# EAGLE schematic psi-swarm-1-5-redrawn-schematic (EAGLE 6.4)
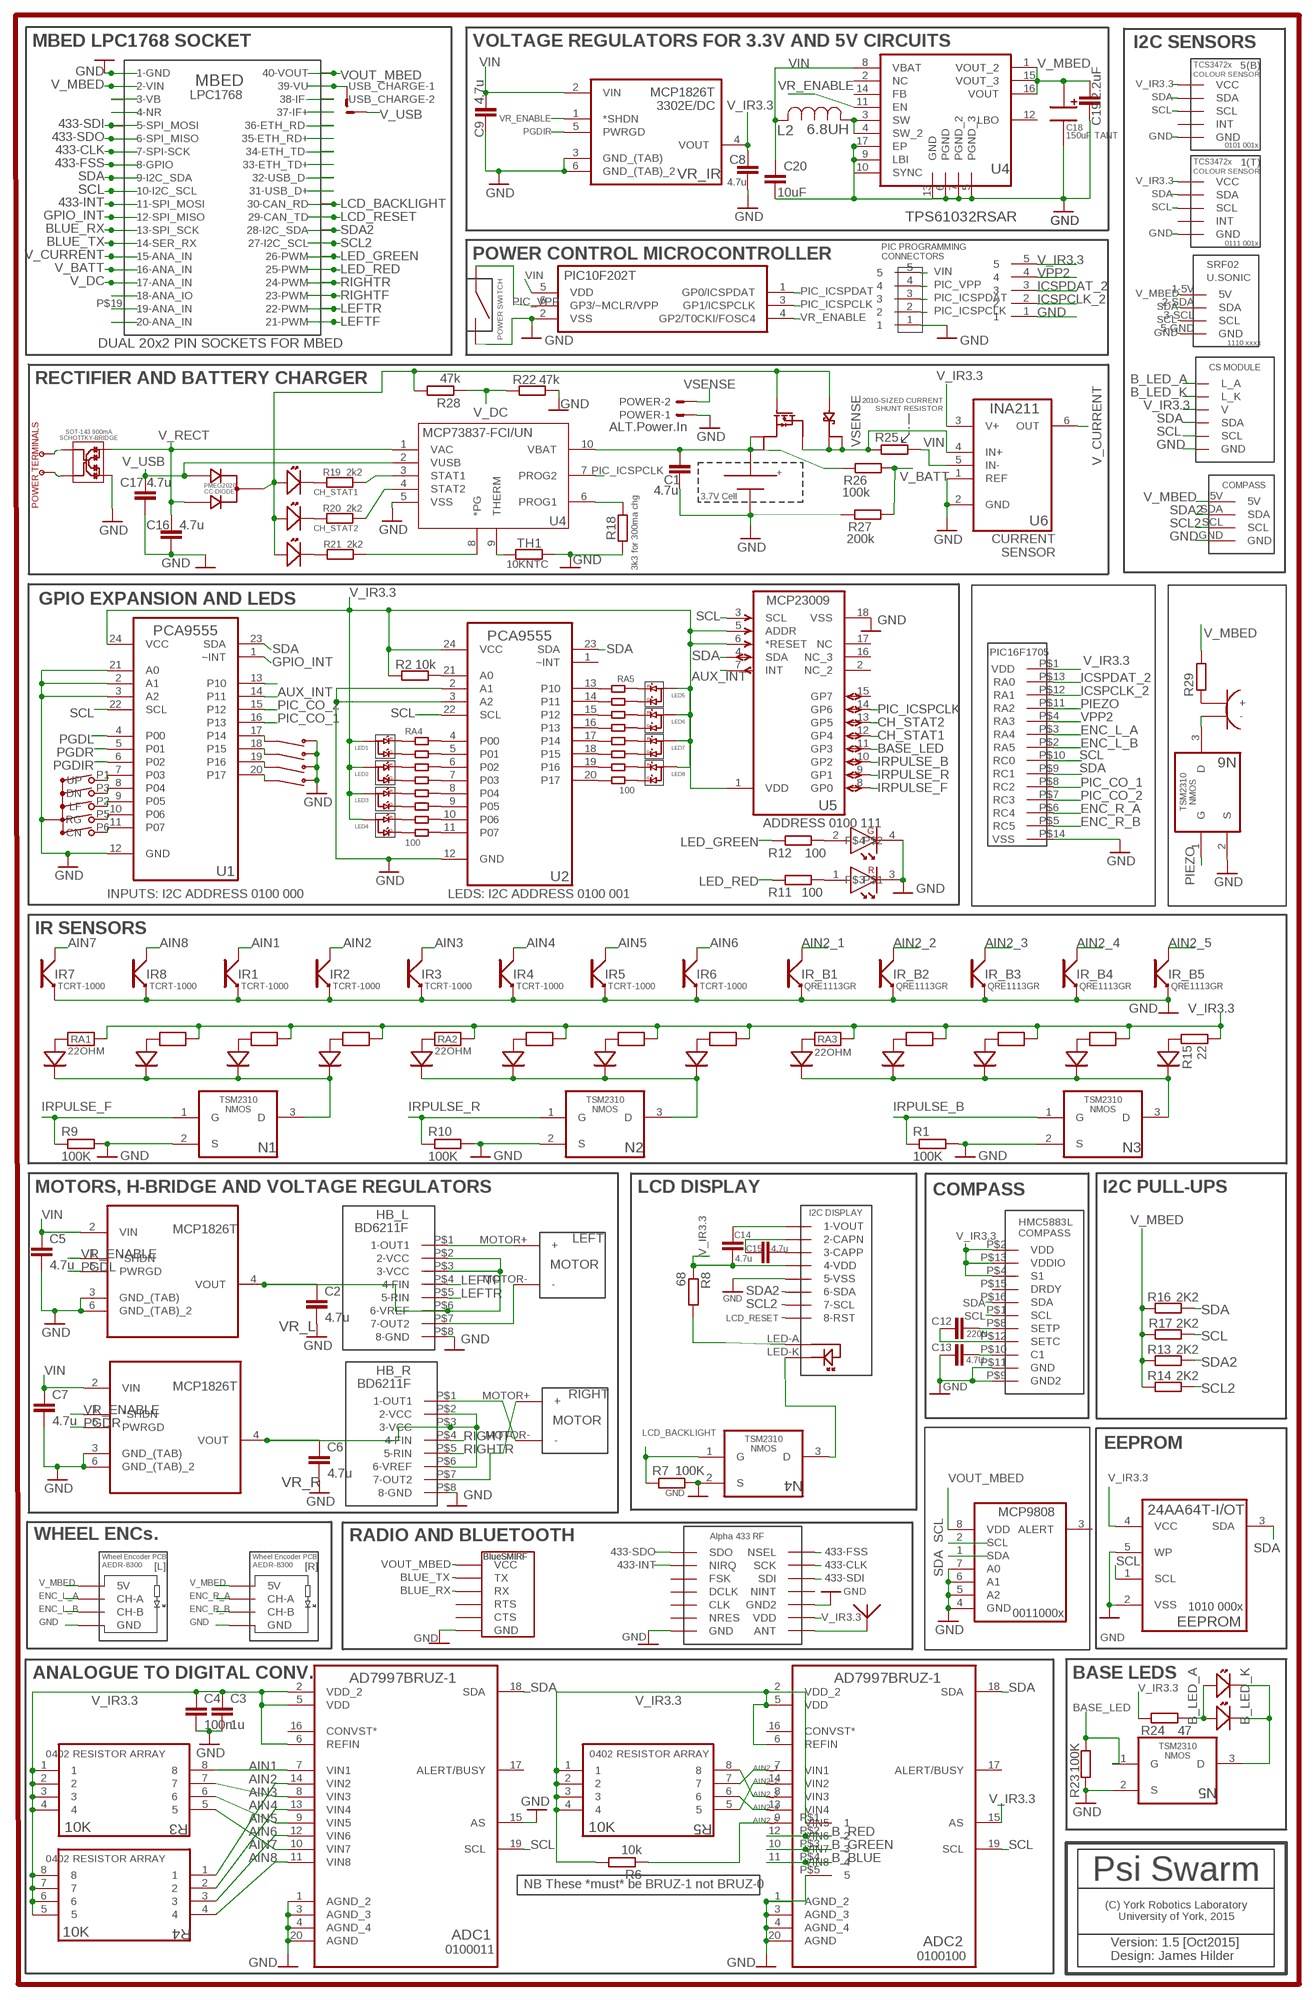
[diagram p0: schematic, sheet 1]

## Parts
ADC1  AD7997BRUZ-1  [SOP65P640X120-20N]
ADC2  AD7997BRUZ-1  [SOP65P640X120-20N]
C1  4.7u  C-EUC1206  [C1206]
C2  4.7u  C-EUC0805  [C0805]
C3  1u  C-EUC0603  [C0603]
C4  100n  C-EUC0603  [C0603]
C5  4.7u  C-EUC0805  [C0805]
C6  4.7u  C-EUC0805  [C0805]
C7  4.7u  C-EUC0805  [C0805]
C8  4.7u  C-EUC0805  [C0805]
C9  4.7u  C-EUC0805  [C0805]
C12  220N  C-EUC0603  [C0603]
C13  4.7U  C-EUC0603  [C0603]
C14  4.7u  C-EUC0805  [C0805]
C15  4.7u  C-EUC0805  [C0805]
C16  4.7u  C-EUC1206  [C1206]
C17  4.7u  C-EUC1206  [C1206]
C18  150uF TANT  2917-TANTALUM-CAP  [2917TANTALUM]
C19  2.2uF  C-EUC0805  [C0805]
C20  10uF  C-EUC0805  [C0805]
EEPROM  24AA64T-I/OT  [SOT95P270X145-5N]
HB_L  HBRIDGE-BD6211FE2-1716259  [ROHM-BD6211]
HB_R  HBRIDGE-BD6211FE2-1716259  [ROHM-BD6211]
IR1  TCRT-1000  [TCRT-1000]
IR2  TCRT-1000  [TCRT-1000]
IR3  TCRT-1000  [TCRT-1000]
IR4  TCRT-1000  [TCRT-1000]
IR5  TCRT-1000  [TCRT-1000]
IR6  TCRT-1000  [TCRT-1000]
IR7  TCRT-1000  [TCRT-1000]
IR8  TCRT-1000  [TCRT-1000]
IR_B1  QRE1113GR-1471020  [QRE1113GR-1471020]
IR_B2  QRE1113GR-1471020  [QRE1113GR-1471020]
IR_B3  QRE1113GR-1471020  [QRE1113GR-1471020]
IR_B4  QRE1113GR-1471020  [QRE1113GR-1471020]
IR_B5  QRE1113GR-1471020  [QRE1113GR-1471020]
L2  6.8UH  ELL8TP6R8NB-8TP  [IND_ELL8TP]
LED1  KPBA3010-DUAL-LED  [KINGBRIGHT-KPBA3010]
LED2  KPBA3010-DUAL-LED  [KINGBRIGHT-KPBA3010]
LED3  KPBA3010-DUAL-LED  [KINGBRIGHT-KPBA3010]
LED4  KPBA3010-DUAL-LED  [KINGBRIGHT-KPBA3010]
LED5  KPBA3010-DUAL-LED  [KINGBRIGHT-KPBA3010]
LED6  KPBA3010-DUAL-LED  [KINGBRIGHT-KPBA3010]
LED7  KPBA3010-DUAL-LED  [KINGBRIGHT-KPBA3010]
LED8  KPBA3010-DUAL-LED  [KINGBRIGHT-KPBA3010]
LED9  2322113-WURTH-DUALLED  [2322113-DUAL-LED-WURTH1411]
LED10  01-ROBOT_KINGBRIGHT-KP-2012-2290331-2335811-2335796  [01-ROBOT_LED-SMD]
LED11  01-ROBOT_KINGBRIGHT-KP-2012-2290331-2335811-2335796  [01-ROBOT_LED-SMD]
LEFT_MOTOR  MICROMETALGEARMOTOR12MM  [MICROMETALGEARMOTOR]
N1  01-ROBOT_TSM2310CX  [01-ROBOT_SOT95P280X130-3N]
N2  01-ROBOT_TSM2310CX  [01-ROBOT_SOT95P280X130-3N]
N3  01-ROBOT_TSM2310CX  [01-ROBOT_SOT95P280X130-3N]
N4  01-ROBOT_TSM2310CX  [01-ROBOT_SOT95P280X130-3N]
N5  01-ROBOT_TSM2310CX  [01-ROBOT_SOT95P280X130-3N]
N6  01-ROBOT_TSM2310CX  [01-ROBOT_SOT95P280X130-3N]
PIC  01-ROBOT_PIC10F202T-I/OT  [01-ROBOT_SOT95P270X145-6N]
POWER  ALT.Power.In  22-23-2021  [22-23-2021]
R1  100K  R-EU_R0805  [R0805]
R2  10k  R-EU_R0805  [R0805]
R3  10K  EXB28V103JX  [RESCAXE50P210X110X45-8N]
R4  10K  EXB28V103JX  [RESCAXE50P210X110X45-8N]
R5  10K  EXB28V103JX  [RESCAXE50P210X110X45-8N]
R6  10k  R-EU_R0805  [R0805]
R7  100K  R-EU_R0805  [R0805]
R8  68  R-EU_R0805  [R0805]
R9  100K  R-EU_R0805  [R0805]
R10  100K  R-EU_R0805  [R0805]
R11  100  R-EU_R0805  [R0805]
R12  100  R-EU_R0805  [R0805]
R13  2K2  R-EU_R0603  [R0603]
R14  2K2  R-EU_R0603  [R0603]
R15  22  R-EU_R0805  [R0805]
R16  2K2  R-EU_R0603  [R0603]
R17  2K2  R-EU_R0603  [R0603]
R18  3k3 for 300ma chg  R-EU_R0805  [R0805]
R19  2k2  R-EU_R0603  [R0603]
R20  2k2  R-EU_R0603  [R0603]
R21  2k2  R-EU_R0603  [R0603]
R22  47k  R-EU_R0603  [R0603]
R23  100K  R-EU_R0805  [R0805]
R24  47  R-EU_R0805  [R0805]
R25  R-EU_R2010  [R2010]
R26  100k  R-EU_R0805  [R0805]
R27  200k  R-EU_R0805  [R0805]
R28  47k  R-EU_R0603  [R0603]
R29  R-EU_R0603  [R0603]
RA1  22OHM  VISHAY_CRA12E083-RESISTORARRAY  [VISHAY-CRA12E083-RES_ARRAY]
RA2  22OHM  VISHAY_CRA12E083-RESISTORARRAY  [VISHAY-CRA12E083-RES_ARRAY]
RA3  22OHM  VISHAY_CRA12E083-RESISTORARRAY  [VISHAY-CRA12E083-RES_ARRAY]
RA4  100  BOURNS-1612550-RESISTORARRAY  [BOURNS-4816P]
RA5  100  BOURNS-1612550-RESISTORARRAY  [BOURNS-4816P]
RIGHT_MOTOR  MICROMETALGEARMOTOR12MM  [MICROMETALGEARMOTOR]
SW1  5-WAY-SWITCH  [ALPS-SKQUCAA010]
SW2  4-WAY-DIP-1524007-MCEMR-04-T  [4WAYDIL-MCEMR-04-T]
SW3  1703878-SWITCH  [SWITCH-1703878]
TH1  10KNTC  R-EU_R0805  [R0805]
U1  PCA9555  01-ROBOT_PCA9555DWR  [01-ROBOT_SOIC127P1030X265-24N]
U2  PCA9555  01-ROBOT_PCA9555DWR  [01-ROBOT_SOIC127P1030X265-24N]
U4  TPS61032RSAR  [QFN65P400X400X100-17N]
U5  01-ROBOT_MCP23009-E/SO  [01-ROBOT_SOIC127P1030X265-18N]
U6  INA211  4WHEEL_ROBOT_LIBRARY_INA214AIDCKT  [4WHEEL_ROBOT_LIBRARY_SOT65P210X110-6N]
U$1  01-ROBOT_MBED-LPC1768-DUALSOCKET  [01-ROBOT_MBED-DUALSOCKET]
U$2  AA-14500-KEYSTONE1028-HOLDER  [KEYSTONE-1028-AAHOLDER]
U$3  01-ROBOT_DISPLAY-2218942-MIDAS-MCCOG21605B6W-FPTLWI  [01-ROBOT_MIDAS-MCCOG21605B6W-DISPLAY]
U$4  01-ROBOT_MCP73837-FCI/UN  [01-ROBOT_SOP50P490X110-8N]
U$5  HMC5883L  [HMC5883L]
U$6  POLOLU_LIBRARY_ALPHA433  [POLOLU_LIBRARY_ALPHA433]
U$7  NEW_PSISWARM_LIBRARY_PIC16F1705  [NEW_PSISWARM_LIBRARY_PIC16F1705]
U$8  POLOLU_LIBRARY_ANTENNA  [POLOLU_LIBRARY_2148530-433MHZANTENNA]
U$9  NEW_PSISWARM_LIBRARY_SRF02-MODULE(HOBBYTRONICS)  [NEW_PSISWARM_LIBRARY_SRF02-MODULE]
U$10  01-ROBOT_BLUESMIRF-HOBBYTRONICS  [01-ROBOT_BLUESMIRF-MODULE]
U$11  01-ROBOT_1859909-PMEG2020CPA-CCDIODE  [01-ROBOT_PMEG2020CPA-CCDIODE-1859909]
U$12  EXPORTED_LIBRARYPSI-SWARM-V13_01-ROBOT_KINGBRIGHT-KP-2012-2290331-2335811-2335796  [EXPORTED_LIBRARYPSI-SWARM-V13_01-ROBOT_LED-SMD]
U$13  EXPORTED_LIBRARYPSI-SWARM-V13_01-ROBOT_KINGBRIGHT-KP-2012-2290331-2335811-2335796  [EXPORTED_LIBRARYPSI-SWARM-V13_01-ROBOT_LED-SMD]
U$14  EXPORTED_LIBRARYPSI-SWARM-V13_01-ROBOT_KINGBRIGHT-KP-2012-2290331-2335811-2335796  [EXPORTED_LIBRARYPSI-SWARM-V13_01-ROBOT_LED-SMD]
U$15  2191755-MOSFET-SCHOTTKY  [2191755-PMFPB8032XP-MOSFET-SCHOTTKY]
U$16  EXPORTED_LIBRARYPSI-SWARM-V13_01-ROBOT_POWER-TERMS  [EXPORTED_LIBRARYPSI-SWARM-V13_01-ROBOT_P-TERMINALS]
U$17  01-ROBOT_1791469-SCHOTTKYBRIDGE  [01-ROBOT_1791469-SCHOTTKY-BRIDGE]
U$18  7857746(RS)-COLOUR-SENSOR  [TCS34725FNCOLOURSENSOR]
U$19  5-PIN-CON  [5-PIN-2MM]
U$20  7857746(RS)-COLOUR-SENSOR  [TCS34725FNCOLOURSENSOR]
U$21  WHEEL-ENCODER-LEFT  [WHEEL-ENCODER]
U$22  WHEEL-ENCODER-RIGHT  [WHEEL-ENCODER-RIGHT]
U$23  POLOLU_LIBRARY_MCP9808-E/MS  [POLOLU_LIBRARY_SOP65P490X110-8N]
U$24  SMT-0540-T-2-R-BUZZERSMT  [SMT-0540-T-2-RBUZZER]
U$25  5-PIN-0.5PITCH  [1.27MMPITCH5PIN]
U$26  COLOUR_SENSOR_CONNECTOR  [COLOUR_SENSOR_MODULE]
U$27  5-PIN-CON  [5-PIN-2MM]
U$28  CMPS11-TILT-COMP-COMPASS  [TILT-COMP-COMPASS-MODULE]
USB_CHARGE  87758-0216  [87758-0216]
VR_IR  01-ROBOT_MCP1826T-3302E/DC  [01-ROBOT_SOT230P700X180-6N]
VR_L  01-ROBOT_MCP1826T-3302E/DC  [01-ROBOT_SOT230P700X180-6N]
VR_R  01-ROBOT_MCP1826T-3302E/DC  [01-ROBOT_SOT230P700X180-6N]

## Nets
433-CLK: U$1.P$7(7-SPI-SCK) U$1.P$47 U$6.13-SCLK(SCK)
433-FSS: U$1.P$8(8-GPIO) U$1.P$48 U$6.14-NSEL(NSEL)
433-INT: U$1.P$11(11-SPI_MOSI) U$1.P$51 U$6.2-NIRQ(NIRQ)
433-SDI: U$1.P$5(5-SPI_MOSI) U$1.P$45 U$6.12-SDI(SDI)
433-SDO: U$1.P$6(6-SPI_MISO) U$1.P$46 U$6.1-SDO(SDO)
AIN1: ADC1.7(VIN1) IR1.COLLECTOR R3.8
AIN2: ADC1.14(VIN2) IR2.COLLECTOR R4.1
AIN2_1: ADC2.7(VIN1) IR_B1.P3-COLLECTOR(COLLECTOR) R5.7
AIN2_2: ADC2.14(VIN2) IR_B2.P3-COLLECTOR(COLLECTOR) R5.5
AIN2_3: ADC2.8(VIN3) IR_B3.P3-COLLECTOR(COLLECTOR) R5.8
AIN2_4: ADC2.13(VIN4) IR_B4.P3-COLLECTOR(COLLECTOR) R5.6
AIN2_5: ADC2.9(VIN5) IR_B5.P3-COLLECTOR(COLLECTOR) R6.1
AIN3: ADC1.8(VIN3) IR3.COLLECTOR R3.7
AIN4: ADC1.13(VIN4) IR4.COLLECTOR R4.2
AIN5: ADC1.9(VIN5) IR5.COLLECTOR R3.6
AIN6: ADC1.12(VIN6) IR6.COLLECTOR R4.3
AIN7: ADC1.10(VIN7) IR7.COLLECTOR R3.5
AIN8: ADC1.11(VIN8) IR8.COLLECTOR R4.4
AUX_INT: U1.14(P11) U5.7(INT)
B_BLUE: ADC2.11(VIN8) U$25.P$4
B_GREEN: ADC2.10(VIN7) U$25.P$3
B_LED_A: LED10.AN LED11.AN R24.1 U$26.LED_A(L_A)
B_LED_K: LED10.CA LED11.CA N5.3(D) U$26.LED_K(L_K)
B_RED: ADC2.12(VIN6) U$25.P$2
BASE_LED: N5.1(G) R23.1 U5.11(GP3)
BLUE_RX: U$1.P$13(13-SPI_SCK) U$1.P$53 U$10.RX
BLUE_TX: U$1.P$14(14-SER_RX) U$1.P$54 U$10.TX
CH_STAT1: R19.2 U5.12(GP4) U$4.3(STAT1)
CH_STAT2: R20.2 U5.13(GP5) U$4.4(STAT2)
ENC_L_A: U$7.P$3(RA4) U$21.CHA(CH-A)
ENC_L_B: U$7.P$2(RA5) U$21.CHB(CH-B)
ENC_R_A: U$7.P$6(RC4) U$22.CHA(CH-A)
ENC_R_B: U$7.P$5(RC5) U$22.CHB(CH-B)
GND: ADC1.1(AGND_2) ADC1.3(AGND_3) ADC1.4(AGND_4) ADC1.15(AS) ADC1.20(AGND) ADC2.1(AGND_2) ADC2.3(AGND_3) ADC2.4(AGND_4) ADC2.20(AGND) C1.2 C2.2 C3.2 C4.2 C5.2 C6.2 C7.2 C8.2 C9.2 C13.1 C16.2 C17.2 C18.CATHODE C19.2 C20.1 EEPROM.2(VSS) EEPROM.5(WP) HB_L.P$8(8-GND) HB_R.P$8(8-GND) IR1.EMITTER IR2.EMITTER IR3.EMITTER IR4.EMITTER IR5.EMITTER IR6.EMITTER IR7.EMITTER IR8.EMITTER IR_B1.P4-EMITTER(EMITTER) IR_B2.P4-EMITTER(EMITTER) IR_B3.P4-EMITTER(EMITTER) IR_B4.P4-EMITTER(EMITTER) IR_B5.P4-EMITTER(EMITTER) LED9.3 LED9.4 N1.2(S) N2.2(S) N3.2(S) N4.2(S) N5.2(S) N6.2(S) PIC.2(VSS) POWER.1 R1.2 R7.2 R9.2 R10.2 R18.1 R22.1 R23.2 R27.2 SW1.P4(C) SW2.5 SW2.6 SW2.7 SW2.8 SW3.2 TH1.1 U1.2(A1) U1.3(A2) U1.12(GND) U1.21(A0) U2.2(A1) U2.3(A2) U2.12(GND) U4.5(PGND_3) U4.6(PGND) U4.7(PGND_2) U4.9(LBI) U4.10(SYNC) U4.13(GND) U4.17(EP) U5.18(VSS) U6.1(REF) U6.2(GND) U$1.P$1(1-GND) U$1.P$41 U$2.- U$3.5-VSS U$4.5(VSS) U$5.P$9(GND2) U$5.P$11(GND) U$6.7-GND(GND) U$6.10-GND(GND2) U$7.P$14(VSS) U$9.5-GND(GND) U$10.GND U$17.1(1-) U$18.3-GND(GND) U$19.1 U$20.3-GND(GND) U$21.GND U$22.GND U$23.4(GND) U$23.5(A2) U$23.6(A1) U$23.7(A0) U$25.P$5 U$26.GND U$27.1 U$28.GND VR_IR.3(GND_(TAB)) VR_IR.6(GND_(TAB)_2) VR_L.3(GND_(TAB)) VR_L.6(GND_(TAB)_2) VR_R.3(GND_(TAB)) VR_R.6(GND_(TAB)_2)
GPIO_INT: U1.1(~INT) U$1.P$12(12-SPI_MISO) U$1.P$52
ICSPCLK_2: U$7.P$12(RA1) U$27.2
ICSPDAT_2: U$7.P$13(RA0) U$27.3
IRPULSE_B: N3.1(G) R1.1 U5.10(GP2)
IRPULSE_F: N1.1(G) R9.1 U5.8(GP0)
IRPULSE_R: N2.1(G) R10.1 U5.9(GP1)
LCD_BACKLIGHT: N4.1(G) R7.1 U$1.P$30(30-CAN_RD) U$1.P$70
LCD_RESET: U$1.P$29(29-CAN_TD) U$1.P$69 U$3.8-RST
LED_GREEN: R12.2 U$1.P$26(26-PWM) U$1.P$66
LED_RED: R11.2 U$1.P$25(25-PWM) U$1.P$65
LEFTF: HB_L.P$4(4-FIN) U$1.P$21(21-PWM) U$1.P$61
LEFTR: HB_L.P$5(5-RIN) U$1.P$22(22-PWM) U$1.P$62
N$1: C12.1 U$5.P$12(SETC)
N$2: C15.2 U$3.3-CAPP
N$3: U$1.P$3(3-VB) U$1.P$43
N$4: U$1.P$4(4-NR) U$1.P$44
N$5: C15.1 U$3.2-CAPN
N$6: N6.3(D) U$24.-
N$7: N4.3(D) U$3.LED-K
N$8: C14.1 U$3.1-VOUT
N$9: U$6.8-ANT(ANT) U$8.ANT
N$10: R8.2 U$3.LED-A
N$11: LED9.1 R11.1
N$12: U1.13(P10)
N$13: R18.2 U$4.6(PROG1)
N$14: R28.2 U$11.P$3 U$12.AN U$13.AN U$14.AN U$15.1(1-A) U$15.5(5-G)
N$16: R29.1 U$24.+
N$18: U$1.P$18(18-ANA_IO) U$1.P$58
N$19: U$1.P$19(19-ANA_IN) U$1.P$59
N$20: U$1.P$20(20-ANA_IN) U$1.P$60
N$21: R19.1 U$12.CA
N$22: U$1.P$39(39-VU) U$1.P$79 USB_CHARGE.1
N$23: U$1.P$38(38-IF-) U$1.P$78
N$24: U$1.P$37(37-IF+) U$1.P$77
N$25: U$1.P$36(36-ETH_RD-) U$1.P$76
N$26: U$1.P$35(35-ETH_RD+) U$1.P$75
N$27: U$1.P$34(34-ETH_TD-) U$1.P$74
N$28: U$1.P$33(33-ETH_TD+) U$1.P$73
N$29: U$1.P$32(32-USB_D-) U$1.P$72
N$30: U$1.P$31(31-USB_D+) U$1.P$71
N$31: LED9.2 R12.1
N$32: R20.1 U$13.CA
N$33: R21.1 U$14.CA
N$34: C12.2 U$5.P$8(SETP)
N$35: C13.2 U$5.P$10(C1)
N$36: R21.2 U$4.8(*PG)
N$37: U$16.P$1 U$17.2
N$38: U$16.P$2 U$17.3
N$39: IR3.CATHODE IR4.CATHODE IR5.CATHODE IR6.CATHODE N2.3(D)
N$40: IR_B1.P1-ANODE(ANODE) RA3.1A
N$41: C1.1 R26.2 U$2.+ U$4.10(VBAT) U$15.3(3-D) U$15.8(8-D)
N$42: TH1.2 U$4.9(THERM)
N$43: HB_L.P$1(1-OUT1) LEFT_MOTOR.MOTOR+(+)
N$44: HB_L.P$7(7-OUT2) LEFT_MOTOR.MOTOR-(-)
N$46: IR1.ANODE RA1.3A
N$47: IR2.ANODE RA1.4A
N$48: IR3.ANODE RA2.1A
N$49: IR4.ANODE RA2.2A
N$50: IR5.ANODE RA2.3A
N$51: IR6.ANODE RA2.4A
N$52: IR7.ANODE RA1.1A
N$53: IR8.ANODE RA1.2A
N$54: IR1.CATHODE IR2.CATHODE IR7.CATHODE IR8.CATHODE N1.3(D)
N$55: IR_B2.P1-ANODE(ANODE) RA3.2A
N$56: IR_B3.P1-ANODE(ANODE) RA3.3A
N$57: IR_B4.P1-ANODE(ANODE) RA3.4A
N$58: IR_B5.P1-ANODE(ANODE) R15.1
N$59: IR_B1.P2-CATHODE(CATHODE) IR_B2.P2-CATHODE(CATHODE) IR_B3.P2-CATHODE(CATHODE) IR_B4.P2-CATHODE(CATHODE) IR_B5.P2-CATHODE(CATHODE) N3.3(D)
N$60: SW1.P1(UP) U1.7(P03)
N$61: SW1.P3(DN) U1.8(P04)
N$62: SW1.P2(LF) U1.9(P05)
N$63: SW1.P5(RG) U1.10(P06)
N$64: SW1.P6(CN) U1.11(P07)
N$65: R2.1 U2.21(A0)
N$67: RA4.9 U2.11(P07)
N$68: RA4.10 U2.10(P06)
N$69: RA4.11 U2.9(P05)
N$70: RA4.12 U2.8(P04)
N$71: RA4.13 U2.7(P03)
N$72: RA4.14 U2.6(P02)
N$73: RA4.15 U2.5(P01)
N$74: RA4.16 U2.4(P00)
N$75: RA5.9 U2.20(P17)
N$76: RA5.10 U2.19(P16)
N$77: RA5.11 U2.18(P15)
N$78: RA5.12 U2.17(P14)
N$79: RA5.13 U2.16(P13)
N$80: RA5.14 U2.15(P12)
N$81: RA5.15 U2.14(P11)
N$82: RA5.16 U2.13(P10)
N$83: SW2.1 U1.20(P17)
N$84: SW2.2 U1.19(P16)
N$85: SW2.3 U1.18(P15)
N$86: SW2.4 U1.17(P14)
N$87: LED1.P2-CRED(CATHODE-RED) RA4.1
N$88: LED1.P3-CGREEN(CATHODE-GREEN) RA4.2
N$90: LED2.P2-CRED(CATHODE-RED) RA4.3
N$91: LED2.P3-CGREEN(CATHODE-GREEN) RA4.4
N$92: LED3.P2-CRED(CATHODE-RED) RA4.5
N$93: LED3.P3-CGREEN(CATHODE-GREEN) RA4.6
N$94: LED4.P2-CRED(CATHODE-RED) RA4.7
N$95: LED4.P3-CGREEN(CATHODE-GREEN) RA4.8
N$96: LED5.P2-CRED(CATHODE-RED) RA5.1
N$97: LED5.P3-CGREEN(CATHODE-GREEN) RA5.2
N$98: LED6.P2-CRED(CATHODE-RED) RA5.3
N$99: LED6.P3-CGREEN(CATHODE-GREEN) RA5.4
N$100: LED7.P2-CRED(CATHODE-RED) RA5.5
N$101: LED7.P3-CGREEN(CATHODE-GREEN) RA5.6
N$102: LED8.P2-CRED(CATHODE-RED) RA5.7
N$103: LED8.P3-CGREEN(CATHODE-GREEN) RA5.8
N$104: HB_R.P$1(1-OUT1) RIGHT_MOTOR.MOTOR-(-)
N$105: C6.1 HB_R.P$2(2-VCC) HB_R.P$3(3-VCC) HB_R.P$6(6-VREF) VR_R.4(VOUT)
N$107: HB_R.P$7(7-OUT2) RIGHT_MOTOR.MOTOR+(+)
N$108: C2.1 HB_L.P$2(2-VCC) HB_L.P$3(3-VCC) HB_L.P$6(6-VREF) VR_L.4(VOUT)
N$109: L2.1 U4.3(SW) U4.4(SW_2)
PGDIR: U1.6(P02) VR_IR.5(PWRGD)
PGDL: U1.4(P00) VR_L.5(PWRGD)
PGDR: U1.5(P01) VR_R.5(PWRGD)
PIC_CO_1: U1.16(P13) U$7.P$8(RC2)
PIC_CO_2: U1.15(P12) U$7.P$7(RC3)
PIC_ICSPCLK: PIC.3(GP1/ICSPCLK) U5.14(GP6) U$4.7(PROG2) U$19.2
PIC_ICSPDAT: PIC.1(GP0/ICSPDAT) U$19.3
PIC_VPP: PIC.6(GP3/~MCLR/VPP) SW3.1 U$19.4
PIEZO: N6.1(G) U$7.P$11(RA2)
RIGHTF: HB_R.P$4(4-FIN) U$1.P$23(23-PWM) U$1.P$63
RIGHTR: HB_R.P$5(5-RIN) U$1.P$24(24-PWM) U$1.P$64
SCL: ADC1.19(SCL) ADC2.19(SCL) EEPROM.1(SCL) R17.2 U1.22(SCL) U2.22(SCL) U5.3(SCL) U$1.P$10(10-I2C_SCL) U$1.P$50 U$5.P$1(SCL) U$7.P$10(RC0) U$9.3-SCL(SCL) U$18.2-SCL(SCL) U$20.2-SCL(SCL) U$23.2(SCL) U$26.SCL
SCL2: R14.1 U$1.P$27(27-I2C_SCL) U$1.P$67 U$3.7-SCL U$28.SCL
SDA: ADC1.18(SDA) ADC2.18(SDA) EEPROM.3(SDA) R16.2 U1.23(SDA) U2.23(SDA) U5.4(SDA) U$1.P$9(9-I2C_SDA) U$1.P$49 U$5.P$16(SDA) U$7.P$9(RC1) U$9.2-SDA(SDA) U$18.6-SDA(SDA) U$20.6-SDA(SDA) U$23.1(SDA) U$26.SDA
SDA2: R13.1 U$1.P$28(28-I2C_SDA) U$1.P$68 U$3.6-SDA U$28.SDA
V_BATT: R26.1 R27.1 U$1.P$16(16-ANA_IN) U$1.P$56
V_CURRENT: U6.6(OUT) U$1.P$15(15-ANA_IN) U$1.P$55
V_DC: R22.2 R28.1 U$1.P$17(17-ANA_IN) U$1.P$57
V_IR3.3: ADC1.2(VDD_2) ADC1.5(VDD) ADC1.6(REFIN) ADC2.2(VDD_2) ADC2.5(VDD) ADC2.6(REFIN) ADC2.15(AS) C3.1 C4.1 C8.1 C14.2 EEPROM.4(VCC) LED1.P1-ANODE(ANODE) LED2.P1-ANODE(ANODE) LED3.P1-ANODE(ANODE) LED4.P1-ANODE(ANODE) LED5.P1-ANODE(ANODE) LED6.P1-ANODE(ANODE) LED7.P1-ANODE(ANODE) LED8.P1-ANODE(ANODE) R2.2 R3.1 R3.2 R3.3 R3.4 R4.5 R4.6 R4.7 R4.8 R5.1 R5.2 R5.3 R5.4 R6.2 R8.1 R15.2 R24.2 RA1.1B RA1.2B RA1.3B RA1.4B RA2.1B RA2.2B RA2.3B RA2.4B RA3.1B RA3.2B RA3.3B RA3.4B U1.24(VCC) U2.24(VCC) U5.1(VDD) U5.5(ADDR) U5.6(*RESET) U6.3(V+) U$3.4-VDD U$5.P$2(VDD) U$5.P$4(S1) U$5.P$13(VDDIO) U$6.9-VDD(VDD) U$7.P$1(VDD) U$18.1-VDD(VCC) U$20.1-VDD(VCC) U$25.P$1 U$26.VDD(V) U$27.5 VR_IR.4(VOUT)
V_MBED: C18.ANODE C19.1 R13.2 R14.2 R16.1 R17.1 R29.2 U4.1(VOUT_2) U4.15(VOUT_3) U4.16(VOUT) U$1.P$2(2-VIN) U$1.P$42 U$9.1-5V(5V) U$21.VCC-5V(5V) U$22.VCC-5V(5V) U$28.5V
V_RECT: C16.1 U$4.1(VAC) U$11.P$2 U$17.4(4+)
V_USB: C17.1 U$4.2(VUSB) U$11.P$1 USB_CHARGE.2
VIN: C5.1 C7.1 C9.1 C20.2 L2.2 PIC.5(VDD) R25.2 U4.8(VBAT) U6.5(IN-) U$19.5 VR_IR.2(VIN) VR_L.2(VIN) VR_R.2(VIN)
VOUT_MBED: U$1.P$40(40-VOUT) U$1.P$80 U$10.VCC U$23.8(VDD)
VPP2: U$7.P$4(RA3) U$27.4
VR_ENABLE: PIC.4(GP2/T0CKI/FOSC4) U4.11(EN) VR_IR.1(*SHDN) VR_L.1(*SHDN) VR_R.1(*SHDN)
VSENSE: POWER.2 R25.1 U6.4(IN+) U$15.4(4-S) U$15.6(6-K) U$15.7(7-K)
Unconnected: ADC1.16(CONVST*) ADC1.17(ALERT/BUSY) ADC2.16(CONVST*) ADC2.17(ALERT/BUSY) U2.1(~INT) U4.2(NC) U4.12(LBO) U4.14(FB) U5.2(NC_2) U5.15(GP7) U5.16(NC_3) U5.17(NC) U$5.P$15(DRDY) U$6.3-FSK(FSK) U$6.4-DCLK(DCLK) U$6.5-CLK(CLK) U$6.6-NRES(NRES) U$6.11-NINT(NINT) U$10.CTS U$10.RTS U$18.5-INT(INT) U$20.5-INT(INT) U$23.3(ALERT)

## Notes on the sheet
- I2C SENSORS
- MBED LPC1768 SOCKET | VOLTAGE REGULATORS FOR 3.3V AND 5V CIRCUITS
- 5(B)
- MCP1826T
  3302E/DC
- 0101 001x
- 1(T)
- 0111 001x
- POWER CONTROL MICROCONTROLLER
- PIC PROGRAMMING
  CONNECTORS
- PIC10F202T
- POWER SWITCH
- 1110 xxxx
- DUAL 20x2 PIN SOCKETS FOR MBED
- RECTIFIER AND BATTERY CHARGER
- 2010-SIZED CURRENT
  SHUNT RESISTOR
- POWER TERMINALS
- MCP73837-FCI/UN
- U4
- CURRENT
  SENSOR
- GPIO EXPANSION AND LEDS
- ADDRESS 0100 111
- INPUTS: I2C ADDRESS 0100 000 | LEDS: I2C ADDRESS 0100 001
- IR SENSORS
- MOTORS, H-BRIDGE AND VOLTAGE REGULATORS | LCD DISPLAY | COMPASS | I2C PULL-UPS
- MCP1826T
- LEFT
- MCP1826T
- RIGHT
- EEPROM
- MCP9808
- WHEEL ENCs. | RADIO AND BLUETOOTH
- [L] | [R]
- 1010 000x
- 0011000x
- ANALOGUE TO DIGITAL CONV. | BASE LEDS
- 0402 RESISTOR ARRAY | 0402 RESISTOR ARRAY
- 0402 RESISTOR ARRAY
- Psi Swarm
- NB These *must* be BRUZ-1 not BRUZ-0
- (C) York Robotics Laboratory
  University of York, 2015
- 0100011
- 0100100
- Version: 1.5 [Oct2015]
  Design: James Hilder

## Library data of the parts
ADC1 ADC2 = pololu_library:AD7997BRUZ-1: 10BIT ADC, 8CH I2C I/F, SMD; MPN: AD7997BRUZ-1; OC_FARNELL: 1078305; OC_NEWARK: 31M4429; PACKAGE: TSSOP-20; SUPPLIER: Analog Devices
C1 C2 C5-C9 C14-C17 C19 C20 = rcl:C-EU: CAPACITOR, European symbol
C3 C4 C12 C13 = resistor:C-EU: CAPACITOR, European symbol
C18 = new_5v_reg:2917-TANTALUM-CAP
EEPROM = 01-robot:24AA64T-I/OT: 64K I2C Serial EEPROM ,SOT23-5; MPN: 24AA64T-I/OT; OC_FARNELL: 2101260; OC_NEWARK: 08P0062; PACKAGE: SOT23-5; SUPPLIER: MICROCHIP
HB_L HB_R = 01-robot:HBRIDGE-BD6211FE2-1716259
IR1-IR8 = 01-robot:TCRT-1000
IR_B1-IR_B5 = 01-robot:QRE1113GR-1471020
L2 = Panasonic-ELL:ELL: Choke Coils; CURRENTRATING: 3.5A; MPN: ELL8TP6R8NB; OC_FARNELL: 1865671; OC_NEWARK: 56T0936; PACKAGE: SMD; SUPPLIER: PANASONIC
LED1-LED8 = 01-robot:KPBA3010-DUAL-LED
LED9 = 01-robot:2322113-WURTH-DUALLED
LED10 LED11 = EXPORTED_LIBRARYpsi-swarm-v13:01-ROBOT_KINGBRIGHT-KP-2012-2290331-2335811-2335796
LEFT_MOTOR RIGHT_MOTOR = 01-robot:MICROMETALGEARMOTOR12MM
N1-N6 = EXPORTED_LIBRARYpsi-swarm-v13:01-ROBOT_TSM2310CX: 20V N-Channel MOSFET; MPN: TSM2310CX; OC_FARNELL: 1864585; OC_NEWARK: 27T2995; PACKAGE: SOT-23-3; SUPPLIER: TAIWAN SEMICONDUCTOR
PIC = EXPORTED_LIBRARYpsi-swarm-v13:01-ROBOT_PIC10F202T-I/OT: 8-bit Flash Microcontroller; MPN: PIC10F202T-I/OT; OC_FARNELL: 9942874; OC_NEWARK: 07J7310; PACKAGE: SOT-6; SUPPLIER: Microchip Technology
POWER = con-molex:22-23-2021: .100" (2.54mm) Center Header - 2 Pin; MF: MOLEX; MPN: 22-23-2021; OC_FARNELL: 1462926; OC_NEWARK: 25C3832
R1 R2 R7 R9 R10 R15 R19-R21 R23 R24 R29 TH1 = rcl:R-EU_: RESISTOR, European symbol
R3-R5 = Panasonic-EXB-ERJ:EXB28V: Chip Resistor Array; MPN: EXB28V103JX; OC_FARNELL: 2060058; OC_NEWARK: 65T9056; PACKAGE: 0402; POWERRATING: 0.063 W/element; SUPPLIER: PANASONIC; TOLERANCE: ±5 %
R6 R8 R11-R14 R16-R18 R22 R25-R28 = resistor:R-EU_: RESISTOR, European symbol
RA1-RA3 = 01-robot:VISHAY_CRA12E083-RESISTORARRAY
RA4 RA5 = 01-robot:BOURNS-1612550-RESISTORARRAY
SW1 = 01-robot:5-WAY-SWITCH
SW2 = 01-robot:4-WAY-DIP-1524007-MCEMR-04-T
SW3 = pololu_library:1703878-SWITCH
U1 U2 = EXPORTED_LIBRARYpsi-swarm-v13:01-ROBOT_PCA9555DWR: 16-BIT I2C AND SMBus I/O EXPANDER; MPN: PCA9555DWR; OC_FARNELL: 2101298; OC_NEWARK: 63K6068; PACKAGE: SOIC-24; SUPPLIER: Texas Instruments
U4 = new_5v_reg:TPS61032RSAR: SYNCHRONOUS BOOST CONVERTER; MPN: TPS61032RSAR; OC_FARNELL: 1743713; OC_NEWARK: 90H4861; PACKAGE: QFN-16; SUPPLIER: Texas Instruments
U5 = EXPORTED_LIBRARYpsi-swarm-v13:01-ROBOT_MCP23009-E/SO: IC, I/O EXPANDER, 8BIT, 3.4MHZ,; MPN: McP23009-E/SO; OC_FARNELL: 1699841; OC_NEWARK: 04R7659; PACKAGE: SOIC-18; SUPPLIER: Microchip
U6 = EXPORTED_LIBRARYpsi-swarm-v13:4WHEEL_ROBOT_LIBRARY_INA214AIDCKT: CURRENT SHUNT MONITOR; MPN: INA214AIDCKT; OC_FARNELL: 1754262; OC_NEWARK: 05N1041; PACKAGE: SC-70-6; SUPPLIER: Texas Instruments
U$1 = EXPORTED_LIBRARYpsi-swarm-v13:01-ROBOT_MBED-LPC1768-DUALSOCKET
U$2 = 01-robot:AA-14500-KEYSTONE1028-HOLDER
U$3 = PsiSwarm15Librarypsi-swarm-1-5:01-ROBOT_DISPLAY-2218942-MIDAS-MCCOG21605B6W-FPTLWI
U$4 = EXPORTED_LIBRARYpsi-swarm-v13:01-ROBOT_MCP73837-FCI/UN: Battery Charger; DESCRIPTION: BATTERY CHARGER; MPN: MCP73837-FCI/UN; OC_FARNELL: 1675426; OC_NEWARK: 77M3068; PACKAGE: MSOP-8; SUPPLIER: Microchip
U$5 = NEW_PSISWARM_LIBRARY:HMC5883L
U$6 = EXPORTED_LIBRARYpsi-swarm-v13:POLOLU_LIBRARY_ALPHA433
U$7 = EXPORTED_LIBRARYpsi-swarm-v13:NEW_PSISWARM_LIBRARY_PIC16F1705
U$8 = EXPORTED_LIBRARYpsi-swarm-v13:POLOLU_LIBRARY_ANTENNA
U$9 = PsiSwarm15Librarypsi-swarm-1-5:NEW_PSISWARM_LIBRARY_SRF02-MODULE(HOBBYTRONICS)
U$10 = EXPORTED_LIBRARYpsi-swarm-v13:01-ROBOT_BLUESMIRF-HOBBYTRONICS
U$11 = EXPORTED_LIBRARYpsi-swarm-v13:01-ROBOT_1859909-PMEG2020CPA-CCDIODE
U$12-U$14 = PsiSwarm15Librarypsi-swarm-1-5:EXPORTED_LIBRARYPSI-SWARM-V13_01-ROBOT_KINGBRIGHT-KP-2012-2290331-2335811-2335796
U$15 = 01-robot:2191755-MOSFET-SCHOTTKY
U$16 = psi-swarm-1-4:EXPORTED_LIBRARYPSI-SWARM-V13_01-ROBOT_POWER-TERMS
U$17 = EXPORTED_LIBRARYpsi-swarm-v13:01-ROBOT_1791469-SCHOTTKYBRIDGE
U$18 U$20 = NEW_PSISWARM_LIBRARY:7857746(RS)-COLOUR-SENSOR
U$19 U$27 = 01-robot:5-PIN-CON
U$21 = EXPORTED_LIBRARYpsi-swarm-v13:WHEEL-ENCODER-LEFT
U$22 = EXPORTED_LIBRARYpsi-swarm-v13:WHEEL-ENCODER-RIGHT
U$23 = psi-swarm-1-3:POLOLU_LIBRARY_MCP9808-E/MS: Digital Temperature Sensor,MSOP-8; MPN: MCP9808-E/MS; OC_FARNELL: 2080523; OC_NEWARK: 89T8871; PACKAGE: MSOP-8; SUPPLIER: MICROCHIP
U$24 = psi-swarm-1-4:SMT-0540-T-2-R-BUZZER
U$25 = psi-swarm-1-3:5-PIN-0.5PITCH
U$26 = PsiSwarm15Librarypsi-swarm-1-5:COLOUR_SENSOR_CONNECTOR
U$28 = PsiSwarm15Librarypsi-swarm-1-5:CMPS11-TILT-COMP-COMPASS
USB_CHARGE = con-molex:87758-0216: 2 Pin - 2mm Dual Row Single Wafer, Vertical T/H HDR; MPN: 87758-0216; OC_FARNELL: unknown; OC_NEWARK: 94M1513
VR_IR = EXPORTED_LIBRARYpsi-swarm-v13:01-ROBOT_MCP1826T-3302E/DC: IC, LDO, 3.3V, 1A,; MPN: MCP1826T-3302E/DC; OC_FARNELL: 1578429; OC_NEWARK: 08N6499; PACKAGE: SOT223-5; SUPPLIER: Microchip
VR_L VR_R = psi-swarm-1-3:01-ROBOT_MCP1826T-3302E/DC: IC, LDO, 3.3V, 1A,; MPN: MCP1826T-3302E/DC; OC_FARNELL: 1578429; OC_NEWARK: 08N6499; PACKAGE: SOT223-5; SUPPLIER: Microchip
